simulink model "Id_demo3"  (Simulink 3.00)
settings: Solver=ode45  SolverMode=SingleTasking  StartTime=0.0  StopTime=10  RelTol=1e-3  AbsTol=1e-3
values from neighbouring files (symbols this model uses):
  Au = [a0 a1;a2]    [data_id1.m]    (also in data_id2.m = [a0;[a1 a2]])
  Ay = [A0 A1;A2]    [data_id1.m]    (also in data_id2.m = A0)
  Bu = [b0;b1]    [data_id1.m]    (also in data_id2.m)
  By = [B0;B1]    [data_id1.m]    (also in data_id2.m)
  Cu = [c0 c1]/den(1)    [data_id1.m]    (also in data_id2.m = [c0 c1])
  Cy = [C0;C1]/den(1)    [data_id1.m]    (also in data_id2.m = [C0;C1])
  Du = zeros(in*(cit+1),in)    [data_id1.m]    (also in data_id2.m = zeros(cit*in,in))
  Dy = -[zeros(out,out);By]/den(1)    [data_id1.m]    (also in data_id2.m = [D1;D2])

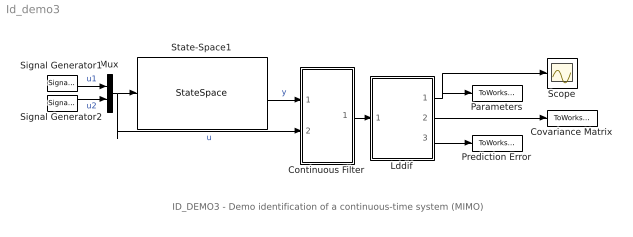
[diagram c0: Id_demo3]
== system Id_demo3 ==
  note: ID_DEMO3 - Demo identification of a continuous-time system (MIMO)
  Continuous Filter : Subsystem  mask(C-Filter){par=[2,2], cit=[0], men=[1], tc=[1]}
      mask prompts: par "No. of inputs and outputs -  [in,out]:"; cit "Numerator degree -  [dn]:"; men "Denominator degree -  [dd]:"; tc "Time constant of the filter - [Tc]:"
      mask help: C-filter: Continuous filters Authors: Lubos Cirka and Miroslav Fikar 1998 - 2004
      mask init:
      | in=par(1); out=par(2);  eval('data_id1');
  Covariance Matrix : ToWorkspace  VariableName=CovMatrix  SampleTime=0  SaveFormat=Matrix
  Lddif : Subsystem  mask(LDDIF){par=[4,2], L=[0.985], d=[0.01], poc=[0 0 0 0 0 0 0 0], kov=[10e6], ts=[1]}
      mask prompts: par "No. of estimated parameters and outputs - [n,m]:"; L "Exponential forgetting - [L]:"; d "Bittanti's correction - [d]:"; poc "Initial parameter estimates - [theta(1) ... theta(n)]:"; kov "Covariance matrix (see help, standard - [10e6]):"; ts "Sampling period - [ts]:"
      mask help: LDDIF: + Bittanti's corrections Authors: Lubos Cirka and Miroslav Fikar 1998 - 2004
      mask init:
      | n=par(1); m=par(2);
  Mux : Mux  Inputs=2
  Parameters : ToWorkspace  VariableName=AB  SampleTime=0  SaveFormat=Matrix
  Prediction Error : ToWorkspace  VariableName=PredError  SampleTime=0  SaveFormat=Matrix
  Scope : Scope
  Signal Generator1 : SignalGenerator  WaveForm=sine  Amplitude=1  Frequency=1  Units=rad/sec
  Signal Generator2 : SignalGenerator  WaveForm=square  Amplitude=1  Frequency=2  Units=rad/sec
  State-Space1 : StateSpace  A=[-23 30;15 -20]  B=[1 1.3;1.1 2.1]  C=[23 -30;-15 20]  D=[0 0;0 0]  X0=0
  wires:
  State-Space1/1 -> Continuous Filter/1(y)  "y"
  Mux/1 -> State-Space1/1, Continuous Filter/2(u)  "u"
  Continuous Filter/1("y, z") -> Lddif/1("y, z")
  Lddif/1(theta) -> Scope/1, Parameters/1
  Lddif/2(covariance matrix) -> Covariance Matrix/1
  Lddif/3(prediction error) -> Prediction Error/1
  Signal Generator1/1 -> Mux/1  "u1"
  Signal Generator2/1 -> Mux/2  "u2"

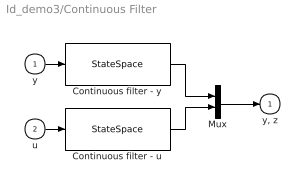
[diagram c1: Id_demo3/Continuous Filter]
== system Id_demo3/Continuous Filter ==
  y : Inport  Port=1  PortWidth=-1  SampleTime=-1  DataType=auto
  u : Inport  Port=2  PortWidth=-1  SampleTime=-1  DataType=auto
  Continuous filter - u : StateSpace  A=Au  B=Bu  C=Cu  D=Du  X0=0
  Continuous filter - y : StateSpace  A=Ay  B=By  C=Cy  D=Dy  X0=0
  Mux : Mux  Inputs=2
  "y, z" : Outport  Port=1  InitialOutput=0
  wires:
  y/1 -> Continuous filter - y/1
  u/1 -> Continuous filter - u/1
  Continuous filter - y/1 -> Mux/1
  Continuous filter - u/1 -> Mux/2
  Mux/1 -> "y, z"/1

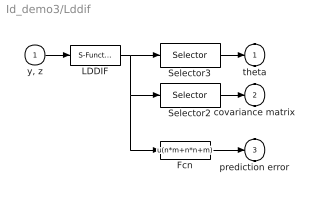
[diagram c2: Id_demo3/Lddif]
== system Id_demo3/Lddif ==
  "y, z" : Inport  Port=1  PortWidth=-1  SampleTime=-1  DataType=auto
  Fcn : Fcn  Expr=u(n*m+n*n+m)
  LDDIF : S-Function  FunctionName=lddif_s  Parameters=m, n, L, d, poc, kov, ts  PortCounts=[]  SFunctionModules=''
  Selector2 : Selector  Elements=[n*m:1:n*m+n*n]  InputPortWidth=n*m+n*n+m
  Selector3 : Selector  Elements=[1:1:n*m]  InputPortWidth=n*m+n*n+m
  theta : Outport  Port=1  InitialOutput=0
  covariance matrix : Outport  Port=2  InitialOutput=0
  prediction error : Outport  Port=3  InitialOutput=0
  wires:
  "y, z"/1 -> LDDIF/1
  LDDIF/1 -> Selector3/1, Selector2/1, Fcn/1
  Selector2/1 -> covariance matrix/1
  Selector3/1 -> theta/1
  Fcn/1 -> prediction error/1
